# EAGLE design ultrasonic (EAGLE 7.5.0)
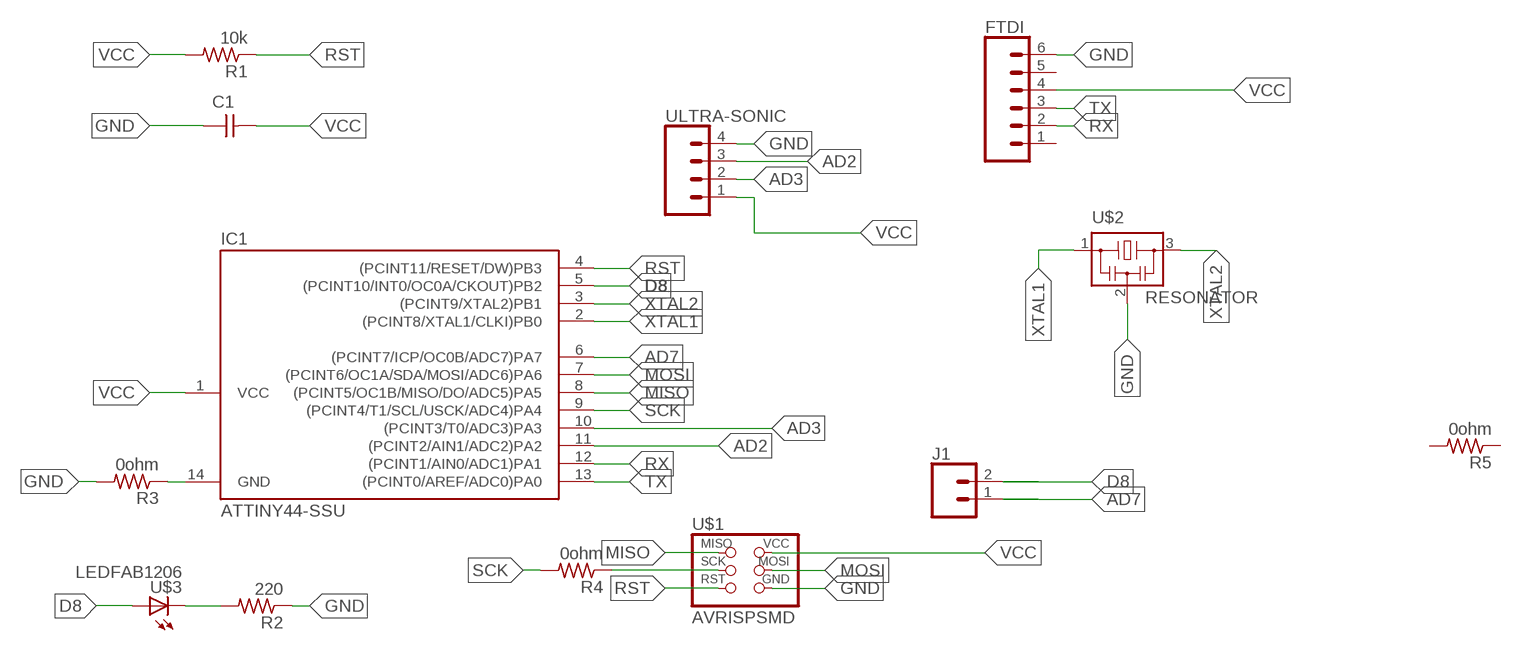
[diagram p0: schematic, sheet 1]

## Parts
C1  CAP-UNPOLARIZEDFAB  [C1206FAB]
FTDI  CONN_06LOCK  [1X06_LOCK]
IC1  ATTINY44-SSU  [SOIC14]
J1  CONN_02  [1X02]
R1  10k  RES-US1206FAB  [R1206FAB]
R2  220  RES-US1206FAB  [R1206FAB]
R3  0ohm  RES-US1206FAB  [R1206FAB]
R4  0ohm  RES-US1206FAB  [R1206FAB]
R5  0ohm  RES-US1206FAB  [R1206FAB]
U$1  AVRISPSMD  [2X03SMD]
U$2  RESONATOR  [EFOBM]
U$3  LEDFAB1206  [LED1206FAB]
ULTRA-SONIC  CONN_04  [1X04]

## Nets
AD2: IC1.11((PCINT2/AIN1/ADC2)PA2) ULTRA-SONIC.3
AD3: IC1.10((PCINT3/T0/ADC3)PA3) ULTRA-SONIC.2
AD7: IC1.6((PCINT7/ICP/OC0B/ADC7)PA7) J1.1
D8: IC1.5((PCINT10/INT0/OC0A/CKOUT)PB2) J1.2 U$3.1(A)
GND: C1.1 FTDI.6 R2.1 R3.2 U$1.6(GND) U$2.2 ULTRA-SONIC.4
MISO: IC1.8((PCINT5/OC1B/MISO/DO/ADC5)PA5) U$1.1(MISO)
MOSI: IC1.7((PCINT6/OC1A/SDA/MOSI/ADC6)PA6) U$1.4(MOSI)
N$1: R2.2 U$3.2(C)
N$2: IC1.14(GND) R3.1
N$3: R4.1 U$1.3(SCK)
RST: IC1.4((PCINT11/RESET/DW)PB3) R1.1 U$1.5(RST)
RX: FTDI.2 IC1.12((PCINT1/AIN0/ADC1)PA1)
SCK: IC1.9((PCINT4/T1/SCL/USCK/ADC4)PA4) R4.2
TX: FTDI.3 IC1.13((PCINT0/AREF/ADC0)PA0)
VCC: C1.2 FTDI.4 IC1.1(VCC) R1.2 U$1.2(VCC) ULTRA-SONIC.1
XTAL1: IC1.2((PCINT8/XTAL1/CLKI)PB0) U$2.1
XTAL2: IC1.3((PCINT9/XTAL2)PB1) U$2.3
Unconnected: FTDI.1 FTDI.5 R5.1 R5.2

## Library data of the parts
C1 = fab:CAP-UNPOLARIZED
FTDI = SparkFun-Connectors:CONN_06: Multi connection point. Often used as Generic Header-pin footprint for 0.1 inch spaced/style header connections On any of the 0.1 inch spaced packages, you can populate with these: Break Away Headers - Straight (PRT-00116) Break Away Male Headers - Right Angle (PRT-00553) Female Headers (PRT-00115)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
IC1 = fab:ATTINY44
J1 = SparkFun-Connectors:CONN_02: Multi connection point. Often used as Generic Header-pin footprint for 0.1 inch spaced/style header connections
R1-R5 = fab:RES-US: Resistor (US Symbol)
U$1 = fab:AVRISP
U$2 = fab:RESONATOR
U$3 = fab:LED: LED
ULTRA-SONIC = SparkFun-Connectors:CONN_04: Multi connection point. Often used as Generic Header-pin footprint for 0.1 inch spaced/style header connections On any of the 0.1 inch spaced packages, you can populate with these: Break Away Headers - Straight (PRT-00116) Break Away Male Headers - Right Angle (PRT-00553) Female Headers (PRT-00115)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; PROD_ID: CONN-09696

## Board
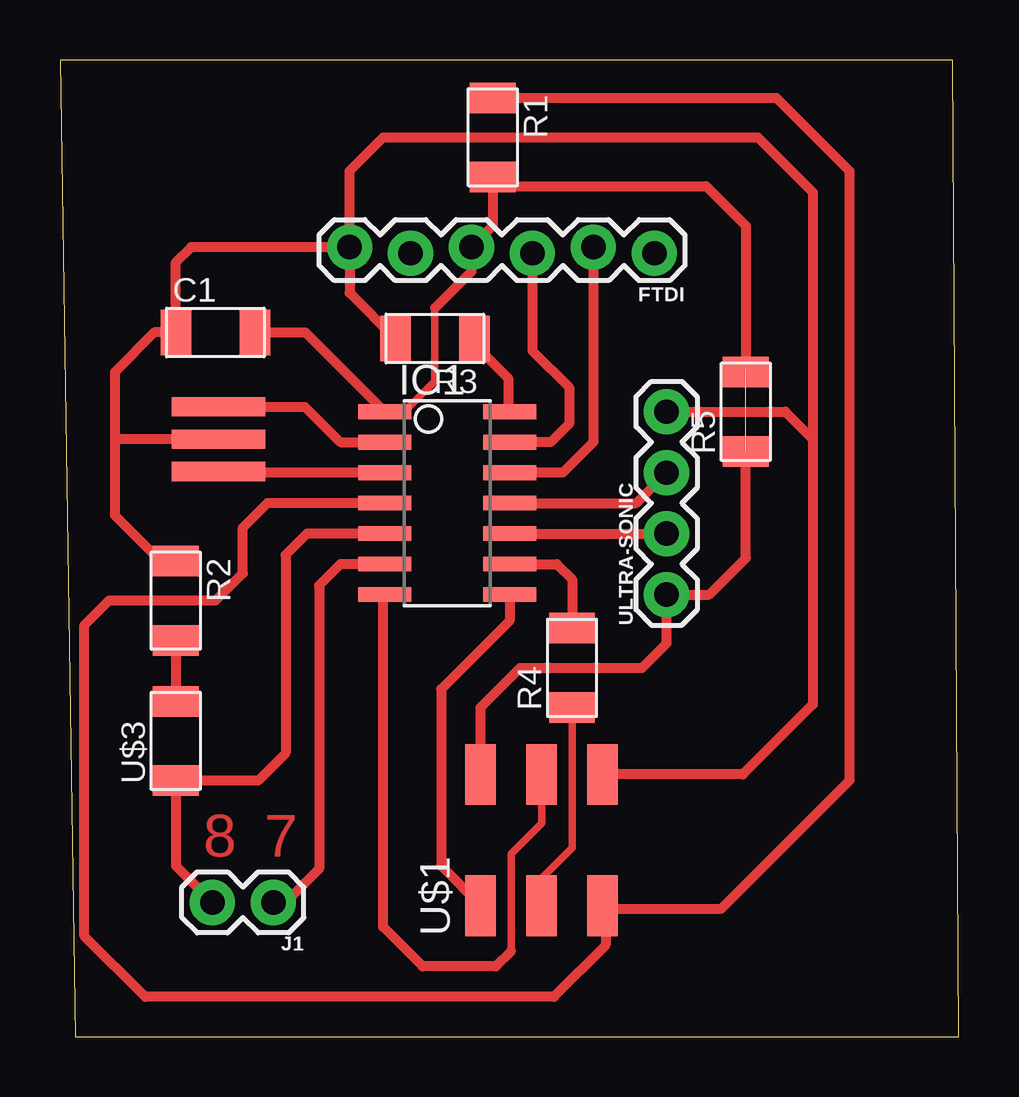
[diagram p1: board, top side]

Size 37.45 x 40.69 mm. Coordinates in mm from the lower left corner, seen from the top.
Outline: 0.64,0 37.45,0 37.19,40.69 0,40.69 0.64,0
Copper layers (1*16): Top 0.035mm / dielectric 1.5mm / Bottom 0.035mm
Design rules "default": minimum track width 10mil, minimum drill 24mil, track to track 8mil, track to pad 8mil, pad to pad 8mil, via to via 8mil, smd to smd 8mil, copper to edge 40mil, drill to drill 8mil, minimum pad ring 10mil, minimum via ring 8mil, stop-mask expansion 4mil, vias tented up to drill 0mil, thermal gap 10mil

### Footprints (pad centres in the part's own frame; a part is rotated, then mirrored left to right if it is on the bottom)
C1206FAB = smd 1.27 x 1.905: 1 -1.651,0; 2 1.651,0
1X06_LOCK = drill 1.016 pad 1.88: 1 0,0; 2 2.54,-0.254; 3 5.08,0; 4 7.62,-0.254; 5 10.16,0; 6 12.7,-0.254
SOIC14 = smd 0.61 x 2.21: 1 -3.81,-2.603; 2 -2.54,-2.603; 3 -1.27,-2.603; 4 0,-2.603; 5 1.27,-2.603; 6 2.54,-2.603; 7 3.81,-2.603; 8 3.81,2.603; 9 2.54,2.603; 10 1.27,2.603; 11 0,2.603; 12 -1.27,2.603; 13 -2.54,2.603; 14 -3.81,2.603
1X02 = drill 1.016 pad 1.88: 1 0,0; 2 2.54,0
R1206FAB = smd 1.27 x 1.905: 1 -1.651,0; 2 1.651,0
2X03SMD = smd 2.54 x 1.27: 1 -2.54,2.54; 2 2.92,2.54; 3 -2.54,0; 4 2.92,0; 5 -2.54,-2.54; 6 2.92,-2.54
EFOBM = smd 0.8 x 3.9: 1 -1.35,0; 2 0,0; 3 1.35,0
LED1206FAB = smd 1.27 x 1.905: 1 -1.651,0; 2 1.651,0
1X04 = drill 1.016 pad 1.88: 1 0,0; 2 2.54,0; 3 5.08,0; 4 7.62,0

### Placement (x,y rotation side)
C1  6.48,29.34 0 top
FTDI  24.77,32.64 180 top
IC1  16.13,22.23 270 top
J1  8.89,5.59 180 top
R1  18.03,37.46 270 top
R2  4.83,18.16 270 top
R3  15.62,29.08 180 top
R4  21.34,15.37 90 top
R5  28.57,26.04 90 top
U$1  20.07,8 90 top
U$2  6.6,24.89 270 top
U$3  4.83,12.32 90 top
ULTRA-SONIC  25.27,18.42 90 top

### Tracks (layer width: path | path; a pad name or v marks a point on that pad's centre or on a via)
AD2
  Top 0.406: IC1.11 24,22.23 ULTRA-SONIC.3
AD3
  Top 0.406: IC1.10 ULTRA-SONIC.2
AD7
  Top 0.406: IC1.6 11.68,19.69 10.79,18.8 10.79,6.98 9.4,5.59 J1.1
D8
  Top 0.406: IC1.5 10.29,20.96 9.4,20.07 9.4,11.81 8.25,10.67 U$3.1 4.83,7.11 J1.2
GND
  Top 0.406: FTDI.6 12.06,36.07 13.46,37.46 29.08,37.46 31.37,35.18 31.37,24.89 | 2.29,24.77 2.29,27.69 3.94,29.34 C1.1 4.83,32.26 5.46,32.89 FTDI.6 | 2.29,24.77 2.29,21.72 4.19,19.81 R2.1 | U$2.2 2.41,24.89 2.29,24.77 | FTDI.6 12.06,30.99 R3.2 | U$1.6 28.45,10.92 31.37,13.84 31.37,24.89 | ULTRA-SONIC.4 30.23,26.04 31.37,24.89
MISO
  Top 0.406: IC1.8 18.73,17.34 15.88,14.48 15.88,7.11 U$1.1
MOSI
  Top 0.305: 18.8,3.56 18.8,7.62 20.07,8.89 U$1.4
  Top 0.406: 18.8,3.56 18.16,2.92 15.11,2.92 13.46,4.57 13.46,18.35 IC1.7
N$1
  Top 0.406: R2.2 U$3.2
N$2
  Top 0.406: R3.1 17.27,28.83 18.67,27.43 18.67,26.1 IC1.14
N$3
  Top 0.305: R4.1 21.34,7.87 20.07,6.6 20.07,6.1
  Top 0.406: 20.07,6.1 U$1.3
RST
  Top 0.406: R1.1 29.84,39.12 32.89,36.07 32.89,10.67 27.56,5.33 22.73,5.33 | 22.73,5.33 U$1.5 | 22.73,5.33 22.73,3.81 20.57,1.65 3.56,1.65 1.02,4.19 1.02,17.15 2.03,18.16 6.48,18.16 7.62,19.3 7.62,21.21 8.64,22.23 IC1.4
RX
  Top 0.406: FTDI.2 22.23,24.77 20.95,23.5 IC1.12
SCK
  Top 0.406: IC1.9 20.7,19.69 21.34,19.05 R4.2
TX
  Top 0.406: FTDI.3 19.68,28.58 21.21,27.05 21.21,25.53 20.45,24.77 IC1.13
VCC  (1 unrouted)
  Top 0.305: IC1.1 14.35,26.04 15.62,27.31 15.62,30.35
  Top 0.406: C1.2 10.22,29.34 IC1.1 | 15.62,30.35 17.14,31.88 FTDI.4 18.03,33.78 R1.2 18.41,35.43 26.92,35.43 28.57,33.78 28.57,27.81 | 28.57,24.38 28.57,19.94 27.05,18.42 ULTRA-SONIC.1 25.27,16.38 24.26,15.37 19.18,15.37 17.53,13.72 U$1.2
XTAL1
  Top 0.406: U$2.1 10.21,26.24 11.68,24.77 IC1.2
XTAL2
  Top 0.406: IC1.3 6.65,23.5 U$2.3

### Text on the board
Top: 8 | 7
